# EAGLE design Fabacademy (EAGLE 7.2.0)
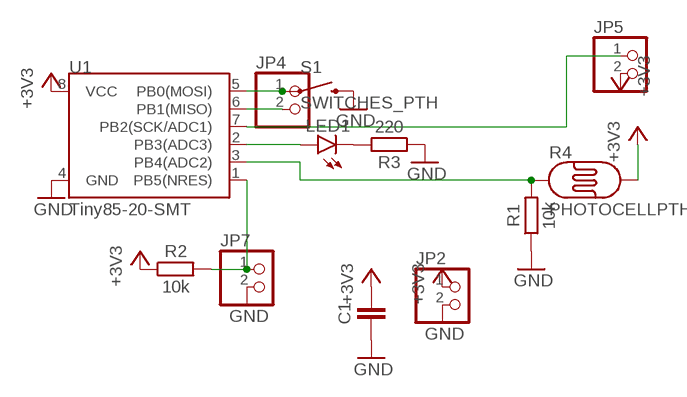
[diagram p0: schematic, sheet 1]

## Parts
C1  CAPACITOR1206  [1206]
JP2  PINHD-1X2  [1X02]
JP4  PINHD-1X2  [1X02]
JP5  PINHD-1X2  [1X02]
JP7  PINHD-1X2  [1X02]
LED1  LED-FKIT-1206  [FKIT-LED-1206]
R1  10k  RESISTOR1206  [1206]
R2  10k  RESISTOR1206  [1206]
R3  220  RESISTOR1206  [1206]
R4  PHOTOCELLPTH  [PHOTOCELL]
S1  SWITCHES_PTH  [TACTILE-PTH]
U1  Tiny85-20-SMT  ATTINY45TINY85-20-SMT  [SO08-EIAJ]

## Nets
+3V3: C1.2 JP2.1 JP5.2 R2.1 R4.2 U1.8(VCC)
GND: C1.1 JP2.2 JP7.2 R1.1 R3.1 S1.3 U1.4(GND)
N$1: R1.2 R4.1 U1.3(PB4(ADC2))
N$2: LED1.A U1.2(PB3(ADC3))
N$3: JP4.1 S1.1 U1.5(PB0(MOSI))
N$4: JP4.2 U1.6(PB1(MISO))
N$5: LED1.C R3.2
N$6: JP5.1 U1.7(PB2(SCK/ADC1))
N$7: JP7.1 R2.2 U1.1(PB5(NRES))

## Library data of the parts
C1 = thar:CAPACITOR
JP2 JP4 JP5 JP7 = pinhead:PINHD-1X2: PIN HEADER
LED1 = SparkFun-LED:LED: LEDs
R1-R3 = thar:RESISTOR
R4 = SparkFun-Sensors:PHOTOCELL: CdS photoresistor. This is a low cost way to detect light levels. Resistance decreases with more incoming light. SparkFun SKU: SEN-09088
S1 = EAGLE_BoosterPack_Library:SWITCHES_: Various NO switches- pushbuttons, reed, etc
U1 = SparkFun-DigitalIC:ATTINY45: Atmel 8-pin 2/4/8kB flash uC; PROD_ID: IC-09092

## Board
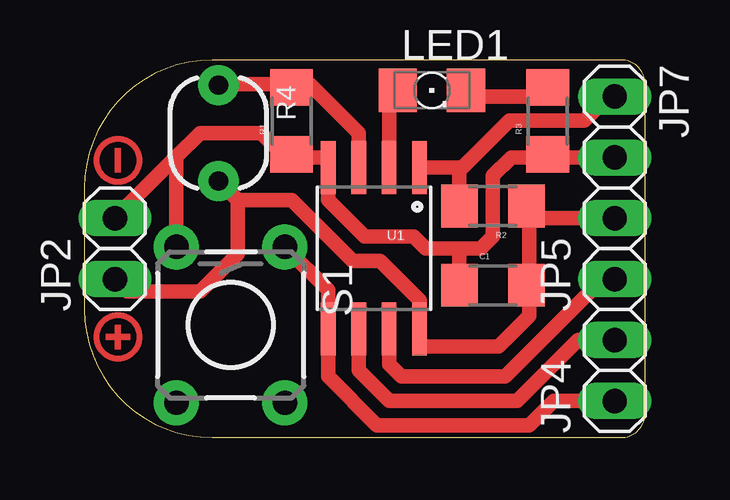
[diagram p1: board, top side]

Size 23.37 x 15.75 mm. Coordinates in mm from the lower left corner, seen from the top.
Outline: 5.33,0 22.35,0 arc90 23.37,1.02 23.37,14.73 arc90 22.35,15.75 5.33,15.75 arc90 0,10.41 0,5.33 arc90 5.33,0
Copper layers (1*16): Top 0.035mm / dielectric 1.5mm / Bottom 0.035mm
Design rules "default": minimum track width 10mil, minimum drill 24mil, track to track 8mil, track to pad 8mil, pad to pad 8mil, via to via 8mil, smd to smd 8mil, copper to edge 40mil, drill to drill 8mil, minimum pad ring 10mil, minimum via ring 8mil, stop-mask expansion 4mil, vias tented up to drill 0mil, thermal gap 10mil

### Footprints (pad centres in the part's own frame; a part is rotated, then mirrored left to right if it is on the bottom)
1206 = smd 1.524 x 1.778: 1 -1.397,0; 2 1.397,0
1X02 = drill 1.016 long: 1 -1.27,0; 2 1.27,0
FKIT-LED-1206 = smd 1.6 x 1.803: A -1.422,0; C 1.422,0
PHOTOCELL = drill 0.8 pad 1.676: 1 -2,0; 2 2,0
TACTILE-PTH = drill 1.016 pad 1.88: 1 -3.251,2.261; 2 3.251,2.261; 3 -3.251,-2.261; 4 3.251,-2.261
SO08-EIAJ = smd 0.61 x 2.21: 1 -1.905,-3.378; 2 -0.635,-3.378; 3 0.635,-3.378; 4 1.905,-3.378; 5 1.905,3.353; 6 0.635,3.353; 7 -0.635,3.353; 8 -1.905,3.353

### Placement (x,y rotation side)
C1  17.02,6.35 0 top
JP2  1.27,7.87 90 top
JP4  22.1,2.79 90 top
JP5  22.1,7.87 90 top
JP7  22.1,12.95 270 top
LED1  14.48,14.48 0 top
R1  8.64,13.21 90 top
R2  17.02,9.65 180 top
R3  19.3,13.21 90 top
R4  5.59,12.7 270 top
S1  6.1,4.7 270 top
U1  12.06,7.87 180 top

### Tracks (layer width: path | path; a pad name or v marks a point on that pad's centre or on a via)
+3V3
  Top 0.61: JP5.2 18.54,9.14 | 18.54,9.14 R2.1 | 18.54,9.14 18.54,6.35 C1.2 18.8,5.84 18.54,5.84 18.54,5.08 17.27,3.81 13.97,3.81 U1.8 13.97,5.71 12.32,7.37 11.18,7.37 8.64,9.91 6.38,9.91 | 6.38,9.91 R4.2 | 6.38,9.91 6.38,7.65 4.83,6.1 1.78,6.1 JP2.1
GND
  Top 0.61: JP7.2 19.3,11.68 | 19.3,11.68 17.78,11.68 17.02,10.92 17.02,8.38 16.51,7.87 15.75,7.87 | 15.75,7.87 14.22,7.87 13.72,8.38 11.68,8.38 10.16,9.91 U1.4 10.16,11.68 9.02,11.68 | C1.1 15.62,7.75 15.75,7.87 | R3.1 19.3,11.68 | 9.02,11.68 R1.1 | 9.02,11.68 8.38,11.68 7.37,12.7 4.83,12.7 3.84,11.71 | 3.84,11.71 JP2.2 | S1.3 3.84,11.71
N$1
  Top 0.61: U1.3 11.43,12.7 9.4,14.73 9.02,14.73 R1.2 8.76,14.61 8.89,14.73 5.56,14.73 R4.1
N$2
  Top 0.61: U1.2 12.7,14.38 LED1.A
N$3
  Top 0.61: JP4.1 19.56,1.52 18.54,0.51 12.19,0.51 10.16,2.54 U1.5 10.16,6.15 S1.1
N$4
  Top 0.61: U1.6 11.43,2.79 12.7,1.52 18.03,1.52 20.57,4.06 JP4.2
N$5
  Top 0.61: R3.2 19.56,14.22 16.15,14.22 LED1.C
N$6
  Top 0.61: U1.7 12.7,3.05 13.21,2.54 17.53,2.54 21.59,6.6 JP5.1
N$7
  Top 0.61: U1.1 15.75,11.25 | R2.2 15.62,11.12 15.75,11.25 | JP7.1 21.84,14.22 20.83,13.21 17.7,13.21 15.75,11.25
(copper drawn outside any net)
  shapes: Top area x3, Top circle x2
